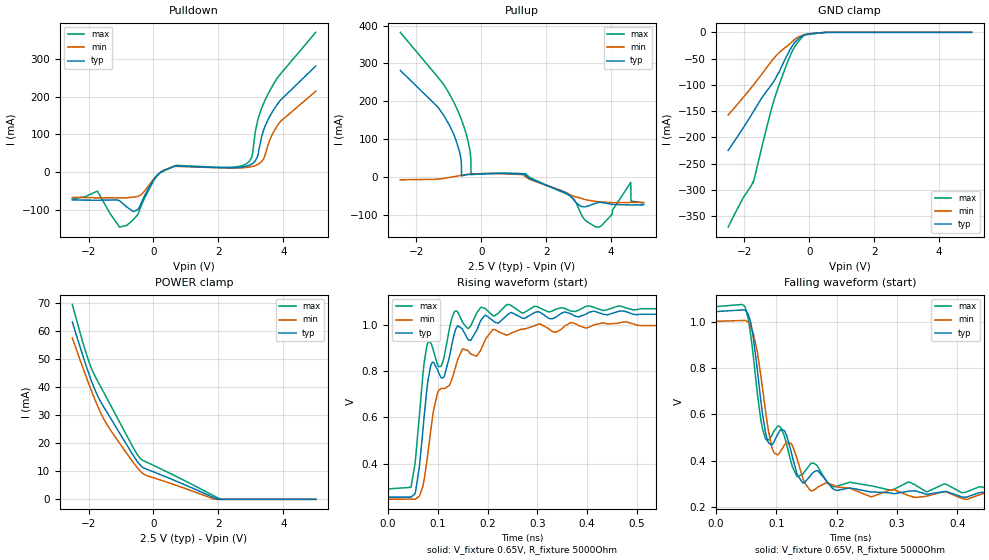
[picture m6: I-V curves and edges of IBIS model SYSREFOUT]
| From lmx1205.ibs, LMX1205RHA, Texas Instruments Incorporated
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|   Model SYSREFOUT
[Model]   SYSREFOUT
Model_type   Output
Polarity   Non-Inverting
Vmeas = 1.25
Vref = 1.25
Cref = 2pF
Rref = 50
|   typ   min   max
C_comp   0.51pF   0.492pF   0.537pF
[Voltage Range]   2.5   2.4   2.6
[Temperature Range]   27   105   -40
[Pullup Reference]   2.5   2.4   2.6
[Pulldown Reference]   -0   0   -0
[Power Clamp Reference]   2.5   2.4   2.6
[GND Clamp Reference]   0   0   0
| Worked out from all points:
|   slope of the pulldown table from 0 to 0.375 V, typ, clamps not added: 13.7 ohm
|   falling waveform, V_fixture 0.65V, R_fixture 5000Ohm: 20-80 % time 63.2ps typ, 66ps min, 61.2ps max; typ from 1.05 V to 0.251 V
|   rising waveform, V_fixture 0.65V, R_fixture 5000Ohm: 20-80 % time 61.5ps typ, 63.4ps min, 22ps max; typ from 0.256 V to 1.04 V
[Pulldown]
|   Voltage   I(typ)   I(min)   I(max)
-2.5V     -73.96mA   -67.38mA   -72mA
-1.728V   -74.89mA   -68.49mA   -50.7mA
-1.038V   -76.63mA   -68.82mA   -146.4mA
-512.5mV  -101.3mA   -65.21mA   -115.9mA
222.5mV   -326.8uA   -224.2uA   -1.219mA
2.848V    15.04mA    12.05mA    21.17mA
3.035V    21.76mA    14.68mA    41.3mA
3.208V    41.5mA     19.89mA    136mA
3.402V    113.4mA    36.21mA    184.1mA
3.567V    145.4mA    81.64mA    213.5mA
3.89V     188.6mA    132.5mA    258.1mA
5V        281.7mA    214.8mA    371.3mA
[GND Clamp]
|   Voltage   I(typ)   I(min)   I(max)
-2.5V     -224.9mA   -157.6mA   -371mA
-2.035V   -182mA     -124mA     -315mA
-1.795V   -158.5mA   -106mA     -293mA
-1.735V   -152.3mA   -101.4mA   -284.7mA
-1.728V   -151.6mA   -100.9mA   -286.9mA
-1.315V   -112.1mA   -67.18mA   -181.9mA
-1.03V    -86.67mA   -45.1mA    -117.8mA
-565mV    -30.06mA   -20.06mA   -41.05mA
-407.5mV  -16.57mA   -11.6mA    -23.65mA
-190mV    -5.981mA   -5.344mA   -7.19mA
545mV     0A         0A         0A
5V        0A         0A         0A
[Pullup]
|   Voltage   I(typ)   I(min)   I(max)
-2.5V     281.7mA    -7.813mA   382.3mA
-850mV    112.1mA    533.9uA    197.7mA
-632.5mV  49.4mA     3.777mA    155.6mA
-610mV    2.531mA    4.101mA    150.5mA
-362.5mV  6.64mA     7.206mA    74.25mA
-317.5mV  6.951mA    7.581mA    5.469mA
1.377V    2.438mA    -710uA     8.027mA
2.735V    -50.07mA   -47.27mA   -50.21mA
3.507V    -70.02mA   -64.76mA   -131.8mA
4.603V    -74.42mA   -67.75mA   -14.51mA
4.61V     -74.42mA   -67.74mA   -63.86mA
5V        -73.9mA    -67.25mA   -69.05mA
[POWER Clamp]
|   Voltage   I(typ)   I(min)   I(max)
-2.5V     63.31mA    57.62mA    69.54mA
-2.125V   49.47mA    45.37mA    54.04mA
-2.005V   45.33mA    41.61mA    49.68mA
-1.885V   41.47mA    37.98mA    46.05mA
-1.735V   37.31mA    33.7mA     42.54mA
-1.472V   31.84mA    27.47mA    36.87mA
-617.5mV  15.59mA    13.08mA    18.34mA
-392.5mV  12.02mA    9.904mA    14.45mA
-197.5mV  10.7mA     8.435mA    13.19mA
1.88V     506.6uA    11.12uA    1.135mA
2.06V     0A         0A         28.85uA
5V        0A         0A         0A
[Ramp]
R_load = 5000
|   typ   min   max
dV/dt_r   0.472973/6.13307e-11   0.453375/6.32014e-11   0.463841/3.14845e-11
dV/dt_f   0.477208/6.29716e-11   0.454983/6.59499e-11   0.4747/6.11123e-11
[Falling Waveform]
V_fixture = 0.65V
V_fixture_min = 0.619V
V_fixture_max = 0.677V
R_fixture = 5000Ohm
C_fixture = 0F
|   Time   V(typ)   V(min)   V(max)
0s        1.046V     1.004V     1.068V
49ps      1.051V     1.007V     1.06V
62ps      930.8mV    949.5mV    849.3mV
82ps      523.1mV    617.2mV    494.9mV
96ps      480.5mV    434.8mV    527.4mV
113ps     530.3mV    465.5mV    508.6mV
134ps     344.6mV    411.9mV    332.7mV
157ps     335.8mV    268.8mV    386.2mV
193ps     279.7mV    295mV      287.1mV
1.25ns    250.7mV    245.4mV    276.6mV
[Rising Waveform]
V_fixture = 0.65V
V_fixture_min = 0.619V
V_fixture_max = 0.677V
R_fixture = 5000Ohm
C_fixture = 0F
|   Time   V(typ)   V(min)   V(max)
0s        256.5mV    247.4mV    292mV
46ps      256.4mV    247.9mV    298.8mV
54ps      270.8mV    247.1mV    397.3mV
78ps      721.6mV    411.6mV    908.5mV
89ps      837.2mV    596.3mV    903.4mV
106ps     773.3mV    724.1mV    819.8mV
136ps     980.2mV    820.1mV    1.059V
210ps     1.018V     978mV      1.039V
306ps     1.052V     1.003V     1.07V
1.25ns    1.045V     1.003V     1.065V
